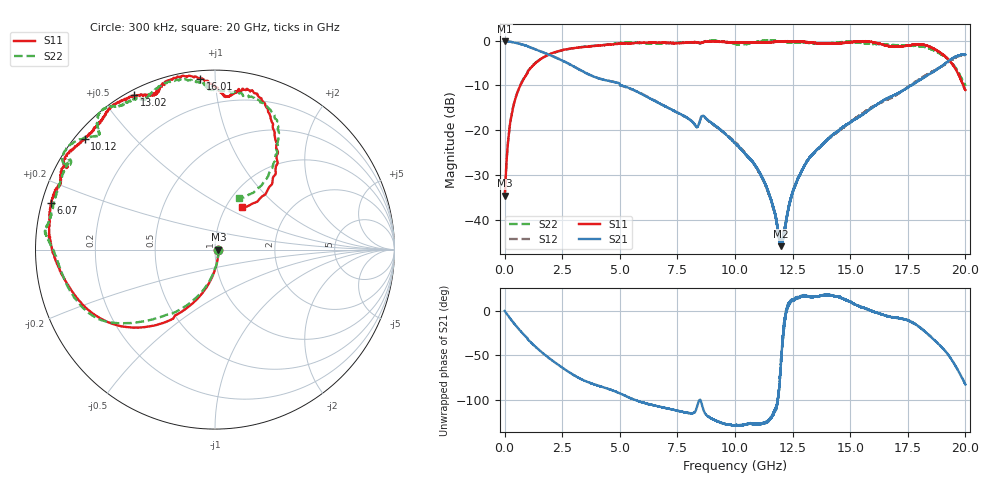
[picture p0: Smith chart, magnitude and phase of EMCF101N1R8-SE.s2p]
!EMCF101N1R8
!Johanson Technology Inc.
!www.johansontechnology.com
!Test Board Conditions:
!Substrate Type  RO4350B
!Substrate Thickness  6.6 mil
!Substrate Dk  3.66
!TL Type: GCPW
!TL Trace Width  13 mil
!TL Gap  7.5 mil
!PART MODE SINGLE ENDED (AKA BYPASS)
!DUT TOPOLOGY	SERIES-SHUNT
# MHz S  dB  R 50
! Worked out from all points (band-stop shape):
!   20001 points, 300 kHz to 20 GHz, reference 50 ohm
!   highest |S21| = -0.16 dB at 3.3 MHz (marker M1); lowest = -45.9 dB at 11.99 GHz (marker M2)
!   |S21| within 3 dB of the highest: start of sweep to 1.928 GHz; 19.85 GHz to end of sweep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
!   lowest |S11| = -34.6 dB at 1.3 MHz (marker M3), VSWR 1.04, Z = 51.9 - j0.0625 ohm
!   |S11| at or under -10 dB: start of sweep to 682.4 MHz; 19.90546 GHz to end of sweep
!   |S22| runs from -34.6 to 0.0 dB; largest |S21 - S12| = 0.022
!   S11 on the Smith chart (normalised r, x): 300 kHz: 1.04, -0.00; 6.07 GHz: 0.03, +0.14; 10.12 GHz: 0.03, +0.37; 13.02 GHz: 0.02, +0.60; 16.01 GHz: 0.04, +0.92; 20 GHz: 1.18, +0.61
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0.3  -34.56 -1.4  -0.17 0.0  -0.16 -0.1  -34.45 -0.3
1.3  -34.60 -1.9  -0.16 -0.0  -0.16 -0.0  -34.62 -1.9
3.3  -34.55 -4.8  -0.16 -0.1  -0.16 -0.1  -34.59 -4.7
300.296  -16.59 -95.2  -0.31 -10.4  -0.30 -10.4  -16.55 -96.6
807.288  -8.75 -116.0  -0.94 -25.8  -0.93 -26.0  -8.65 -118.7
1746.274  -3.55 -139.7  -2.77 -49.4  -2.76 -49.1  -3.57 -141.8
3334.25  -1.49 -166.6  -6.70 -76.9  -6.72 -77.0  -1.43 -166.6
6070.209  -0.44 164.2  -12.25 -103.8  -12.16 -103.5  -0.59 169.8
6667.2  -0.46 160.2  -13.87 -107.6  -13.81 -107.8  -0.59 163.8
8651.17  -0.31 150.7  -16.88 -112.9  -16.88 -113.3  -0.25 150.3
10000.15  -0.39 140.5  -22.89 -128.7  -22.70 -128.4  -0.75 136.4
10122.15  -0.41 139.6  -23.48 -128.7  -23.27 -128.9  -0.81 136.0
11277.13  -0.41 132.1  -31.59 -126.1  -31.79 -126.2  -0.02 130.5
11990.12  -0.15 127.5  -45.89 -60.3  -44.95 -57.5  -0.20 125.1
12493.11  -0.16 122.8  -33.87 11.5  -33.91 12.9  -0.40 122.3
13016.1  -0.25 117.7  -27.95 16.6  -27.83 16.4  -0.42 118.6
13334.1  -0.49 115.0  -25.54 15.6  -25.54 15.2  -0.58 116.1
16010.06  -0.41 94.9  -14.78 -0.9  -14.70 -2.4  -0.73 93.2
16667.05  -1.26 87.1  -12.72 -6.2  -13.07 -6.3  -0.96 92.3
18271.03  -1.07 74.0  -8.01 -23.8  -7.72 -24.1  -1.47 69.3
19310.01  -4.46 54.3  -4.39 -51.4  -4.55 -52.3  -4.46 55.9
20000  -11.05 57.7  -3.13 -82.8  -3.19 -82.2  -10.04 65.3
